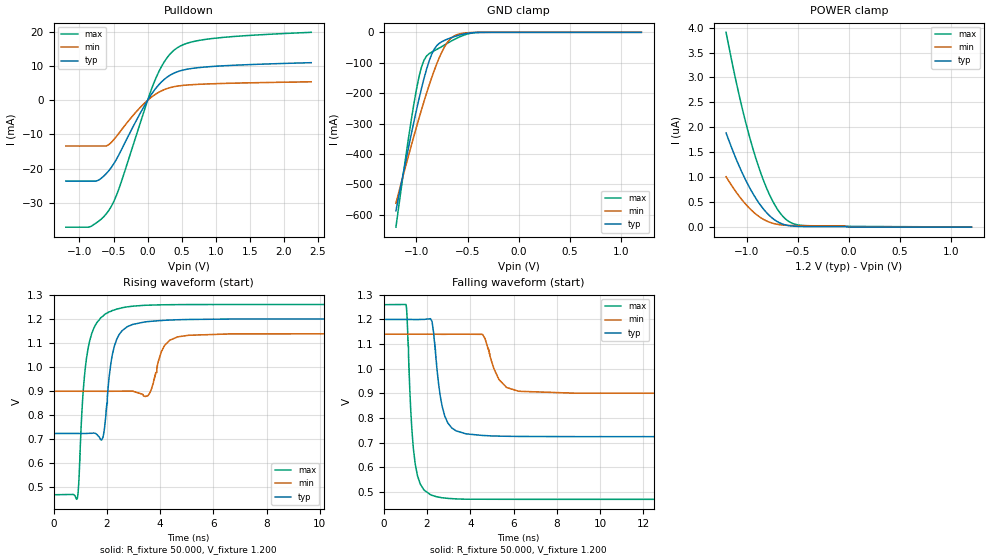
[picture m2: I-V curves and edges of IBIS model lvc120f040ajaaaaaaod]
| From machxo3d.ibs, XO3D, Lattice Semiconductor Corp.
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|   Model lvc120f040ajaaaaaaod
[Model] lvc120f040ajaaaaaaod
Model_type I/O_open_drain
Polarity   Non-Inverting
Enable   Active-Low
Vinl =  0.420V
Vinh =  0.780V
Vmeas =  0.600V
Cref =  0.0F
Rref = 10.00k
Vref = 1.20V
C_comp   4.200pF   3.800pF   7.500pF
[Temperature Range]   25.000   0.105k   -40.000
[Voltage Range]   1.200V   1.140V   1.260V
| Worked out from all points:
|   slope of the pulldown table from 0 to 0.18 V, typ, clamps not added: 36.7 ohm
|   GND clamp passes 1 mA (typ) near -0.44 V on its own axis
|   rising waveform, R_fixture 50.000, V_fixture 1.200: 20-80 % time 361ps typ, 416ps min, 354ps max; typ from 0.724 V to 1.2 V
|   falling waveform, R_fixture 50.000, V_fixture 1.200: 20-80 % time 431ps typ, 632ps min, 307ps max; typ from 1.2 V to 0.724 V
[Pulldown]
|Voltage   I(typ)   I(min)   I(max)
-1.2V     -23.66mA   -13.38mA   -37.14mA
-830mV    -23.66mA   -13.38mA   -36.91mA
-719mV    -23.37mA   -13.38mA   -35.42mA
-534mV    -19.7mA    -12.35mA   -31.11mA
-423mV    -16.01mA   -9.695mA   -26.02mA
-127mV    -4.473mA   -2.488mA   -7.831mA
95mV      2.865mA    1.496mA    5.244mA
243mV     6.106mA    3.121mA    11.23mA
391mV     8.008mA    3.999mA    14.74mA
576mV     9.093mA    4.47mA     16.69mA
909mV     9.852mA    4.817mA    18mA
2.4V      11.02mA    5.419mA    19.91mA
[GND_clamp]
|Voltage   I(typ)   I(min)   I(max)
-1.2V     -586.8mA   -561.6mA   -640.4mA
-1.075V   -375.3mA   -403.2mA   -342.9mA
-1V       -256.8mA   -312.3mA   -188.8mA
-950mV    -184.3mA   -254.5mA   -114.1mA
-925mV    -151.1mA   -226.6mA   -91.28mA
-875mV    -93.98mA   -173.6mA   -70.02mA
-800mV    -43.52mA   -102.9mA   -56.06mA
-725mV    -26.41mA   -48.03mA   -41.59mA
-650mV    -16.51mA   -16.35mA   -27.18mA
-575mV    -8.675mA   -5.014mA   -14.71mA
-375mV    -184.4uA   -82.53uA   -274.8uA
1.2V      0A         0A         0A
[POWER_clamp]
|Voltage   I(typ)   I(min)   I(max)
-1.2V     1.889uA    1.011uA    3.905uA
-1.125V   1.485uA    772.5nA    3.141uA
-1.05V    1.124uA    563.1nA    2.451uA
-975mV    812.1nA    387.4nA    1.845uA
-900mV    550.1nA    247.5nA    1.324uA
-825mV    340.1nA    145.7nA    890.5nA
-750mV    184.9nA    81.62nA    545.5nA
-675mV    85.57nA    49.09nA    292.2nA
-600mV    35.85nA    35.98nA    132.8nA
-525mV    17.84nA    31.28nA    57.78nA
-400mV    11.63nA    28.62nA    28.93nA
1.2V      0A         0A         3.813nA
[Ramp]
| variable   typ   min   max
dV/dt_r   0.286/0.358n   0.144/0.410n   0.476/0.353n
dV/dt_f   0.286/0.431n   0.144/0.602n   0.476/0.308n
R_load = 50.000
[Rising Waveform]
R_fixture= 50.000
V_fixture= 1.200
V_fixture_min= 1.140
V_fixture_max= 1.260
|time   V(typ)   V(min)   V(max)
0s        724mV      899.5mV    469.4mV
895ps     724.1mV    899.5mV    453.8mV
1.124ns   723.9mV    899.5mV    913.5mV
1.298ns   724.4mV    899.5mV    1.078V
1.855ns   707.5mV    899.4mV    1.211V
2.208ns   1.051V     899.4mV    1.235V
3.539ns   1.189V     880.4mV    1.257V
4.169ns   1.194V     1.09V      1.259V
5.069ns   1.198V     1.132V     1.26V
20ns      1.2V       1.14V      1.26V
[Falling Waveform]
R_fixture= 50.000
V_fixture= 1.200
V_fixture_min= 1.140
V_fixture_max= 1.260
|time   V(typ)   V(min)   V(max)
0s        1.2V       1.14V      1.26V
1.037ns   1.2V       1.14V      1.261V
1.249ns   1.2V       1.14V      835.4mV
1.461ns   1.199V     1.14V      611.1mV
2.163ns   1.203V     1.14V      488mV
2.702ns   847.1mV    1.139V     475.6mV
3.344ns   747.5mV    1.14V      471.1mV
4.566ns   728.7mV    1.139V     469.7mV
6.235ns   724.8mV    908.2mV    469.4mV
20ns      724mV      899.5mV    469.4mV
